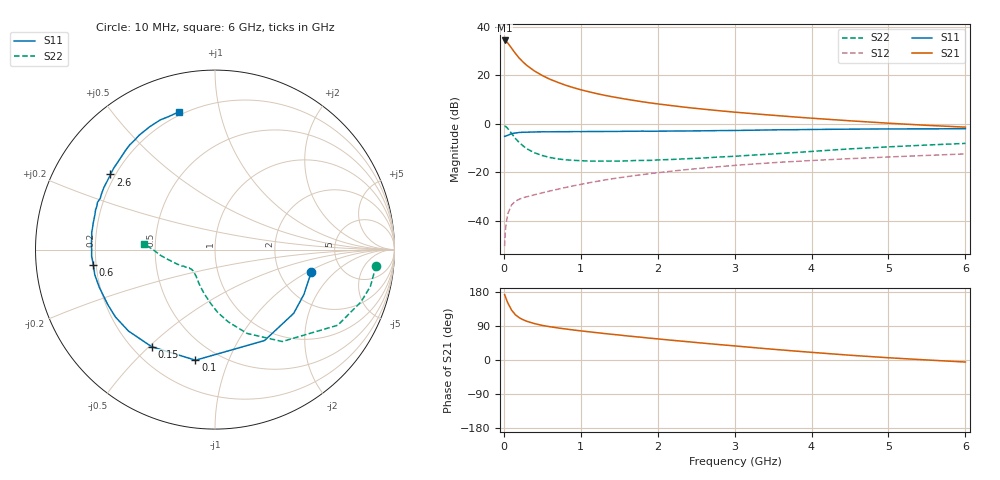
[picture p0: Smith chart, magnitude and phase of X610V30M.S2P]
! SIEMENS Small Signal Semiconductors
! BFP193W
! Si NPN RF Bipolar Junction Transistor in SOT343
! VCE = 10 V  IC = 30 mA
! Common Emitter S-Parameters:  April 1994
# GHz  S  MA  R  50
!  f  S11  S21  S12  S22
! GHz  MAG  ANG  MAG  ANG  MAG  ANG  MAG  ANG
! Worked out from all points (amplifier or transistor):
!   40 points, 10 MHz to 6 GHz, reference 50 ohm
!   highest |S21| = 34.4 dB at 10 MHz (marker M1)
!   |S21| within 3 dB of that: start of sweep to 96.36 MHz
!   unconditionally stable (mu >= 1): 905 MHz to 4.677 GHz
!   at 200 MHz: K = 0.42, MSG = 29.1 dB, |S12| = -31.1 dB
!   at 1.5 GHz: K = 1.10, MAG = 14.5 dB, |S12| = -22.2 dB
!   at 6 GHz: K = 0.95, MSG = 5.5 dB, |S12| = -12.4 dB
!   S11 on the Smith chart (normalised r, x): 10 MHz: 3.04, -1.07; 100 MHz: 0.38, -0.77; 150 MHz: 0.27, -0.51; 600 MHz: 0.19, -0.06; 2.6 GHz: 0.18, +0.31; 6 GHz: 0.18, +0.75
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0.01  0.5511 -12.8  52.26 172.3  0.003 71.5  0.9018 -5.7
0.02  0.5548 -26.7  51.52 167.3  0.0063 72.1  0.8898 -13.3
0.03  0.5642 -39.0  50.3 161.7  0.0087 71.3  0.864 -19.7
0.05  0.577 -61.4  46.51 151.2  0.0138 64.2  0.8036 -31.6
0.1  0.6258 -100.0  36.34 131.9  0.0212 50.8  0.6346 -53.8
0.15  0.6459 -123.1  28.29 119.4  0.0254 44.2  0.5005 -69.0
0.2  0.6621 -136.7  22.62 111.6  0.0278 41.6  0.4101 -79.5
0.25  0.6698 -145.9  18.8 106.2  0.03 40.7  0.3507 -87.5
0.3  0.6714 -152.7  15.9 102.1  0.0313 40.9  0.3047 -94.0
0.4  0.6781 -162.0  12.21 95.9  0.0345 42.6  0.2523 -103.9
0.5  0.6843 -168.2  9.887 91.3  0.0377 44.8  0.2215 -111.5
0.6  0.6831 -173.0  8.276 87.8  0.0412 46.9  0.2018 -117.6
0.8  0.6872 179.7  6.265 81.9  0.0486 50.7  0.1813 -125.8
1.1  0.6933 172.2  4.601 74.6  0.0605 54.0  0.1706 -134.3
1.3  0.6945 167.5  3.898 70.0  0.0689 55.0  0.1702 -137.5
1.6  0.7013 161.6  3.197 63.6  0.0814 55.5  0.1715 -141.2
2.2  0.7093 150.9  2.35 51.8  0.1063 53.9  0.1845 -148.1
2.6  0.7172 144.3  1.999 44.3  0.1227 52.0  0.1973 -152.2
3.2  0.7359 134.8  1.637 33.6  0.1464 48.3  0.2246 -158.6
4.5  0.7753 117.9  1.153 12.6  0.1912 39.7  0.3042 -173.8
5.5  0.7849 109.1  0.93 0.1  0.2229 33.5  0.365 178.1
6  0.7932 104.8  0.853 -5.4  0.2394 31.0  0.3945 175.2
